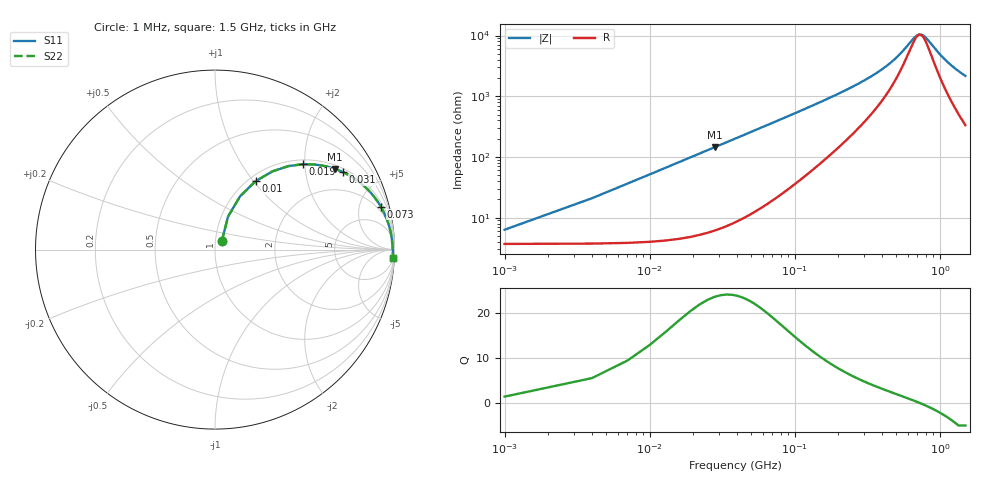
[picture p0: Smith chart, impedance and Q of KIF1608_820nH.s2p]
# MHz S RI R 50
!Freq ReS11 ImS11 ReS21 ImS21 ReS12 ImS12 ReS22 ImS22
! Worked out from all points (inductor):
!   501 points, 1 MHz to 1.5 GHz, reference 50 ohm
!   read as one part in series: L = 819 nH near 7 MHz
!   highest Q = 23.4 at 28 MHz (marker M1), where L = 820 nH
!   self-resonance near 724.6 MHz
!   S11 on the Smith chart (normalised r, x): 1 MHz: 1.07, +0.10; 10 MHz: 1.08, +1.03; 19 MHz: 1.10, +1.96; 31 MHz: 1.13, +3.20; 73 MHz: 1.41, +7.57; 1.5 GHz: 8, -43
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1  0.0381 0.0478  0.9619 -0.0478  0.9619 -0.0478  0.0381 0.0478
4  0.0727 0.1841  0.9273 -0.1841  0.9273 -0.1841  0.0727 0.1841
10  0.2278 0.3823  0.7722 -0.3823  0.7722 -0.3823  0.2278 0.3823
13  0.3208 0.4363  0.6792 -0.4363  0.6792 -0.4363  0.3208 0.4363
19  0.4903 0.4759  0.5097 -0.4759  0.5097 -0.4759  0.4903 0.4759
28  0.6693 0.4497  0.3307 -0.4497  0.3307 -0.4497  0.6693 0.4497
31  0.7111 0.4328  0.2889 -0.4328  0.2889 -0.4328  0.7111 0.4328
40  0.8003 0.3793  0.1997 -0.3793  0.1997 -0.3793  0.8003 0.3793
49  0.8545 0.3311  0.1455 -0.3311  0.1455 -0.3311  0.8545 0.3311
73  0.9237 0.2398  0.0763 -0.2398  0.0763 -0.2398  0.9237 0.2398
106  0.9573 0.1695  0.0427 -0.1695  0.0427 -0.1695  0.9573 0.1695
145  0.9722 0.1236  0.0278 -0.1236  0.0278 -0.1236  0.9722 0.1236
253  0.9842 0.0659  0.0158 -0.0659  0.0158 -0.0659  0.9842 0.0659
502  0.9892 0.0201  0.0108 -0.0201  0.0108 -0.0201  0.9892 0.0201
670  0.9902 0.00425  0.00977 -0.00425  0.00977 -0.00425  0.9902 0.00425
712  0.9904 0.000955  0.00958 -0.000955  0.00958 -0.000955  0.9904 0.000955
751  0.9906 -0.00195  0.00943 0.00195  0.00943 0.00195  0.9906 -0.00195
799  0.9907 -0.00535  0.00926 0.00535  0.00926 0.00535  0.9907 -0.00535
1003  0.9912 -0.0183  0.00882 0.0183  0.00882 0.0183  0.9912 -0.0183
1117  0.9913 -0.0249  0.00874 0.0249  0.00874 0.0249  0.9913 -0.0249
1252  0.9912 -0.0323  0.00877 0.0323  0.00877 0.0323  0.9912 -0.0323
1500  0.9908 -0.045  0.00916 0.045  0.00916 0.045  0.9908 -0.045
